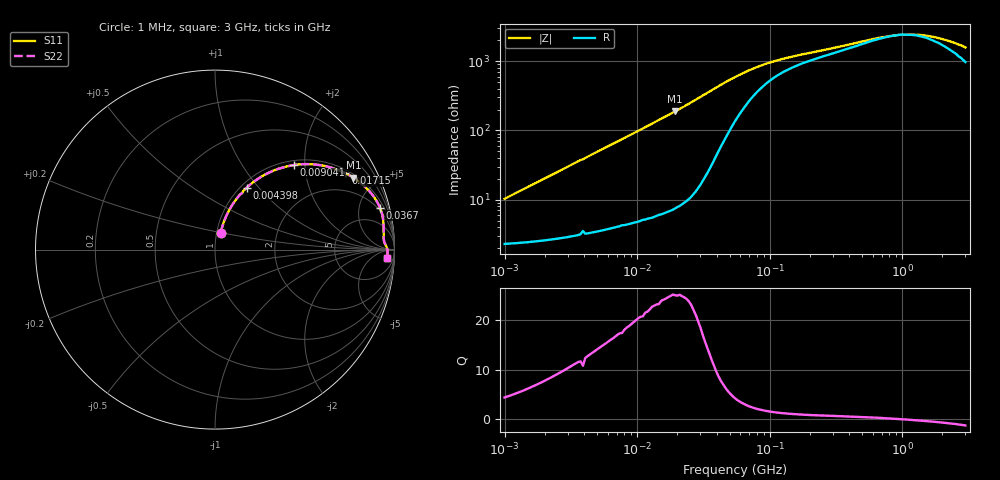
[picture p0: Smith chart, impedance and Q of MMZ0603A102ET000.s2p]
! S-Parameter Data Generated by TDK Corporation
! Copyright(C) 2025 TDK Corporation.
! All Rights Reserved.
! TDK P/N: MMZ0603A102ET000 (Chip Bead)
! Property: |Z|=1000ohm at 100MHz
! Size(LxWxT): 0.6x0.3x0.3mm
! Model Type: s2p (Touchstone File Format Version 1.0)
! Frequency: DC=Yes Start=1MHz Stop=3000MHz 202points Log-sweep
! Model Generated on Feb. 6, 2025
! Terms and conditions regarding TDK Simulation Models:
! 1)This simulation model is being provided solely for informational
!  purposes. Please refer to the specifications of the products in
!  terms of detailed characteristics of such products.
! 2)In no event shall TDK Corporation of any of its subsidiaries be
!  liable for any loss or damage arising, directly or indirectly,
!  from any information contained in this simulation model, including,
!  but not limited to loss or damages arising from any inaccuracies,
!  omissions or errors in connection with such information.
! 3)Any and all copyrights on this simulation model are owned by
!  TDK Corporation.  Duplication or redistribution of this simulation
!  model without prior written permission from TDK Corporation
!  is prohibited.
! 4)This simulation model is subject to any modification or change
!  without any prior notice.
! 5)Neither TDK Corporation nor any of its subsidiaries shall make any
!  warranty, express or implied, including but not limited to the
!  correctness, implied warranties of merchantability and fitness for
!  a particular purpose with respect to this simulation models.
! 6)The use of this simulation model shall be deemed to have consented
!  to the terms and conditions hereof.
! Port Assignments:
!  1 ---@@@--- 2
! Applicable Conditions:
!  Temperature = 25 degC
!  DC Bias Current = 0 A
!  Small Signal Operation
# Hz S MA R 50
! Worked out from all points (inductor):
!   201 points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, 1 MHz to 3 GHz, reference 50 ohm
!   read as one part in series: L = 1.6 uH near 1.041 MHz
!   highest Q = 25.1 at 19.34 MHz (marker M1), where L = 1.55 uH
!   self-resonance near 972.5 MHz
!   S11 on the Smith chart (normalised r, x): 1 MHz: 1.05, +0.20; 4.398 MHz: 1.07, +0.87; 9.041 MHz: 1.09, +1.75; 17.15 MHz: 1.13, +3.32; 36.7 MHz: 1.64, +7.64; 3 GHz: 20, -25
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1000000  0.1004 71.5  0.9728 -5.6  0.9728 -5.6  0.1004 71.5
2226959  0.2133 71.0  0.9521 -12.2  0.9521 -12.2  0.2133 71.0
3900413  0.3475 64.5  0.9062 -20.2  0.9062 -20.2  0.3475 64.5
4398124  0.3873 62.9  0.8929 -22.7  0.8929 -22.7  0.3873 62.9
6305767  0.5108 55.8  0.8285 -30.6  0.8285 -30.6  0.5108 55.8
9040831  0.6426 47.1  0.7336 -39.9  0.7336 -39.9  0.6426 47.1
1.149534e7  0.7265 40.8  0.6543 -46.5  0.6543 -46.5  0.7265 40.8
1.461624e7  0.8 34.5  0.5667 -53.1  0.5667 -53.1  0.8 34.5
1.71545e7  0.8419 30.4  0.5066 -57.3  0.5066 -57.3  0.8419 30.4
1.934349e7  0.8688 27.5  0.4617 -60.2  0.4617 -60.2  0.8688 27.5
2.664524e7  0.9225 20.3  0.3466 -67.1  0.3466 -67.1  0.9225 20.3
3.670325e7  0.9483 14.3  0.2475 -70.9  0.2475 -70.9  0.9483 14.3
5.477226e7  0.9504 9.0  0.1613 -67.6  0.1613 -67.6  0.9504 9.0
7.248696e7  0.9461 6.6  0.1245 -61.1  0.1245 -61.1  0.9461 6.6
9.984923e7  0.9426 4.8  0.09897 -52.2  0.09897 -52.2  0.9426 4.8
1.375402e8  0.942 3.6  0.08364 -44.3  0.08364 -44.3  0.942 3.6
2.136344e8  0.9443 2.5  0.06999 -36.1  0.06999 -36.1  0.9443 2.5
8.005644e8  0.9588 0.3  0.04162 -7.5  0.04162 -7.5  0.9588 0.3
1.147801e9  0.9608 -0.3  0.03957 7.6  0.03957 7.6  0.9608 -0.3
1.519029e9  0.9617 -0.9  0.0411 20.7  0.0411 20.7  0.9617 -0.9
2.177892e9  0.9621 -1.7  0.04807 37.1  0.04807 37.1  0.9621 -1.7
3e9  0.9614 -2.8  0.06087 49.3  0.06087 49.3  0.9614 -2.8
